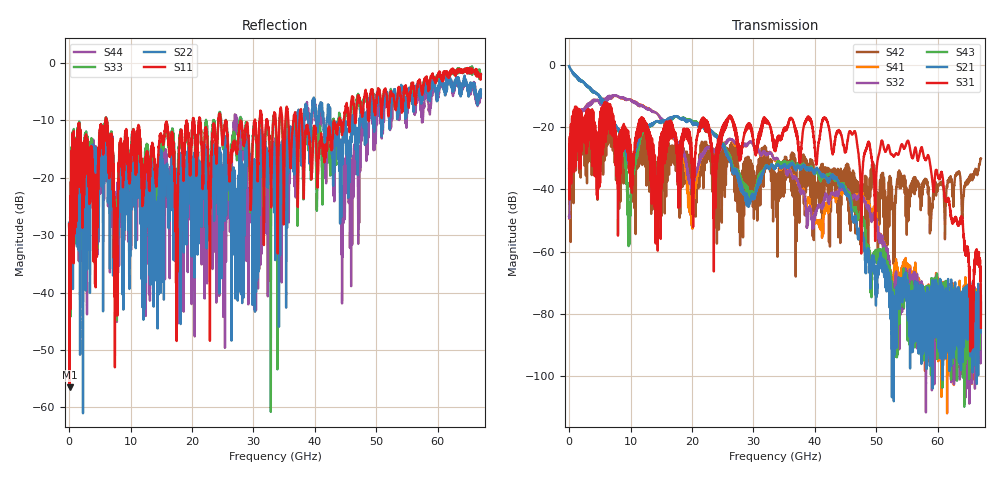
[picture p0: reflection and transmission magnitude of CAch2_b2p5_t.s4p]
!Agilent Technologies,N5247A,US51170199,A.09.90.13
!Agilent N5247A: A.09.90.13
!Date: Tuesday, October 23, 2018 13:28:06
!Correction: S11(Full 4 Port(1,2,3,4))
!S12(Full 4 Port(1,2,3,4))
!S13(Full 4 Port(1,2,3,4))
!S14(Full 4 Port(1,2,3,4))
!S21(Full 4 Port(1,2,3,4))
!S22(Full 4 Port(1,2,3,4))
!S23(Full 4 Port(1,2,3,4))
!S24(Full 4 Port(1,2,3,4))
!S31(Full 4 Port(1,2,3,4))
!S32(Full 4 Port(1,2,3,4))
!S33(Full 4 Port(1,2,3,4))
!S34(Full 4 Port(1,2,3,4))
!S41(Full 4 Port(1,2,3,4))
!S42(Full 4 Port(1,2,3,4))
!S43(Full 4 Port(1,2,3,4))
!S44(Full 4 Port(1,2,3,4))
!S4P File: Measurements: <S11,S12,S13,S14>,
!<S21,S22,S23,S24>,
!<S31,S32,S33,S34>,
!<S41,S42,S43,S44>:
# Hz S  dB  R 50
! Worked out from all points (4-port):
!   6701 points, 10 MHz to 67 GHz, reference 50 ohm
!   strongest paths, dB at 10 MHz, 16.76 GHz, 33.51 GHz, 50.25 GHz, 67 GHz:
!     S31: -33.2, -22.6, -25.7, -30.0, -84.5
!     S21: -0.4, -16.8, -32.9, -64.6, -74.3
!     S43: -0.4, -17.0, -32.7, -61.5, -79.8
!     S32: -48.6, -22.5, -30.4, -52.2, -76.3
!     S41: -48.5, -23.0, -30.8, -51.0, -76.8
!     S42: -33.4, -28.8, -34.6, -63.7, -30.0
!   lowest |S11| = -56.5 dB at 89.99 MHz (marker M1), VSWR 1.00, Z = 50.1 + j0.0507 ohm
!   |S11| at or under -10 dB: start of sweep to 5.98 GHz; 6.103 GHz to 20.15 GHz (14.05 GHz wide, 107 % of centre); 37.88 GHz to 43.98 GHz (6.098 GHz wide, 14.9 % of centre)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
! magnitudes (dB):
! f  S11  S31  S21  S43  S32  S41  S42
! 10 MHz  -28.1  -33.2  -0.4  -0.4  -48.6  -48.5  -33.4
! 89.99 MHz  -56.5  -34.8  -0.8  -0.8  -43.1  -43.0  -35.3
! 7.739 GHz  -35.2  -35.9  -19.8  -20.0  -9.9  -9.9  -34.7
! 19.87 GHz  -14.7  -25.2  -18.3  -17.8  -39.3  -49.6  -32.3
! 43.03 GHz  -10.6  -27.2  -36.2  -36.3  -41.3  -41.8  -34.2
! 55.09 GHz  -5.8  -24.4  -76.9  -70.6  -71.8  -65.9  -50.3
! 67 GHz  -2.0  -84.5  -74.3  -79.8  -76.3  -76.8  -30.0
